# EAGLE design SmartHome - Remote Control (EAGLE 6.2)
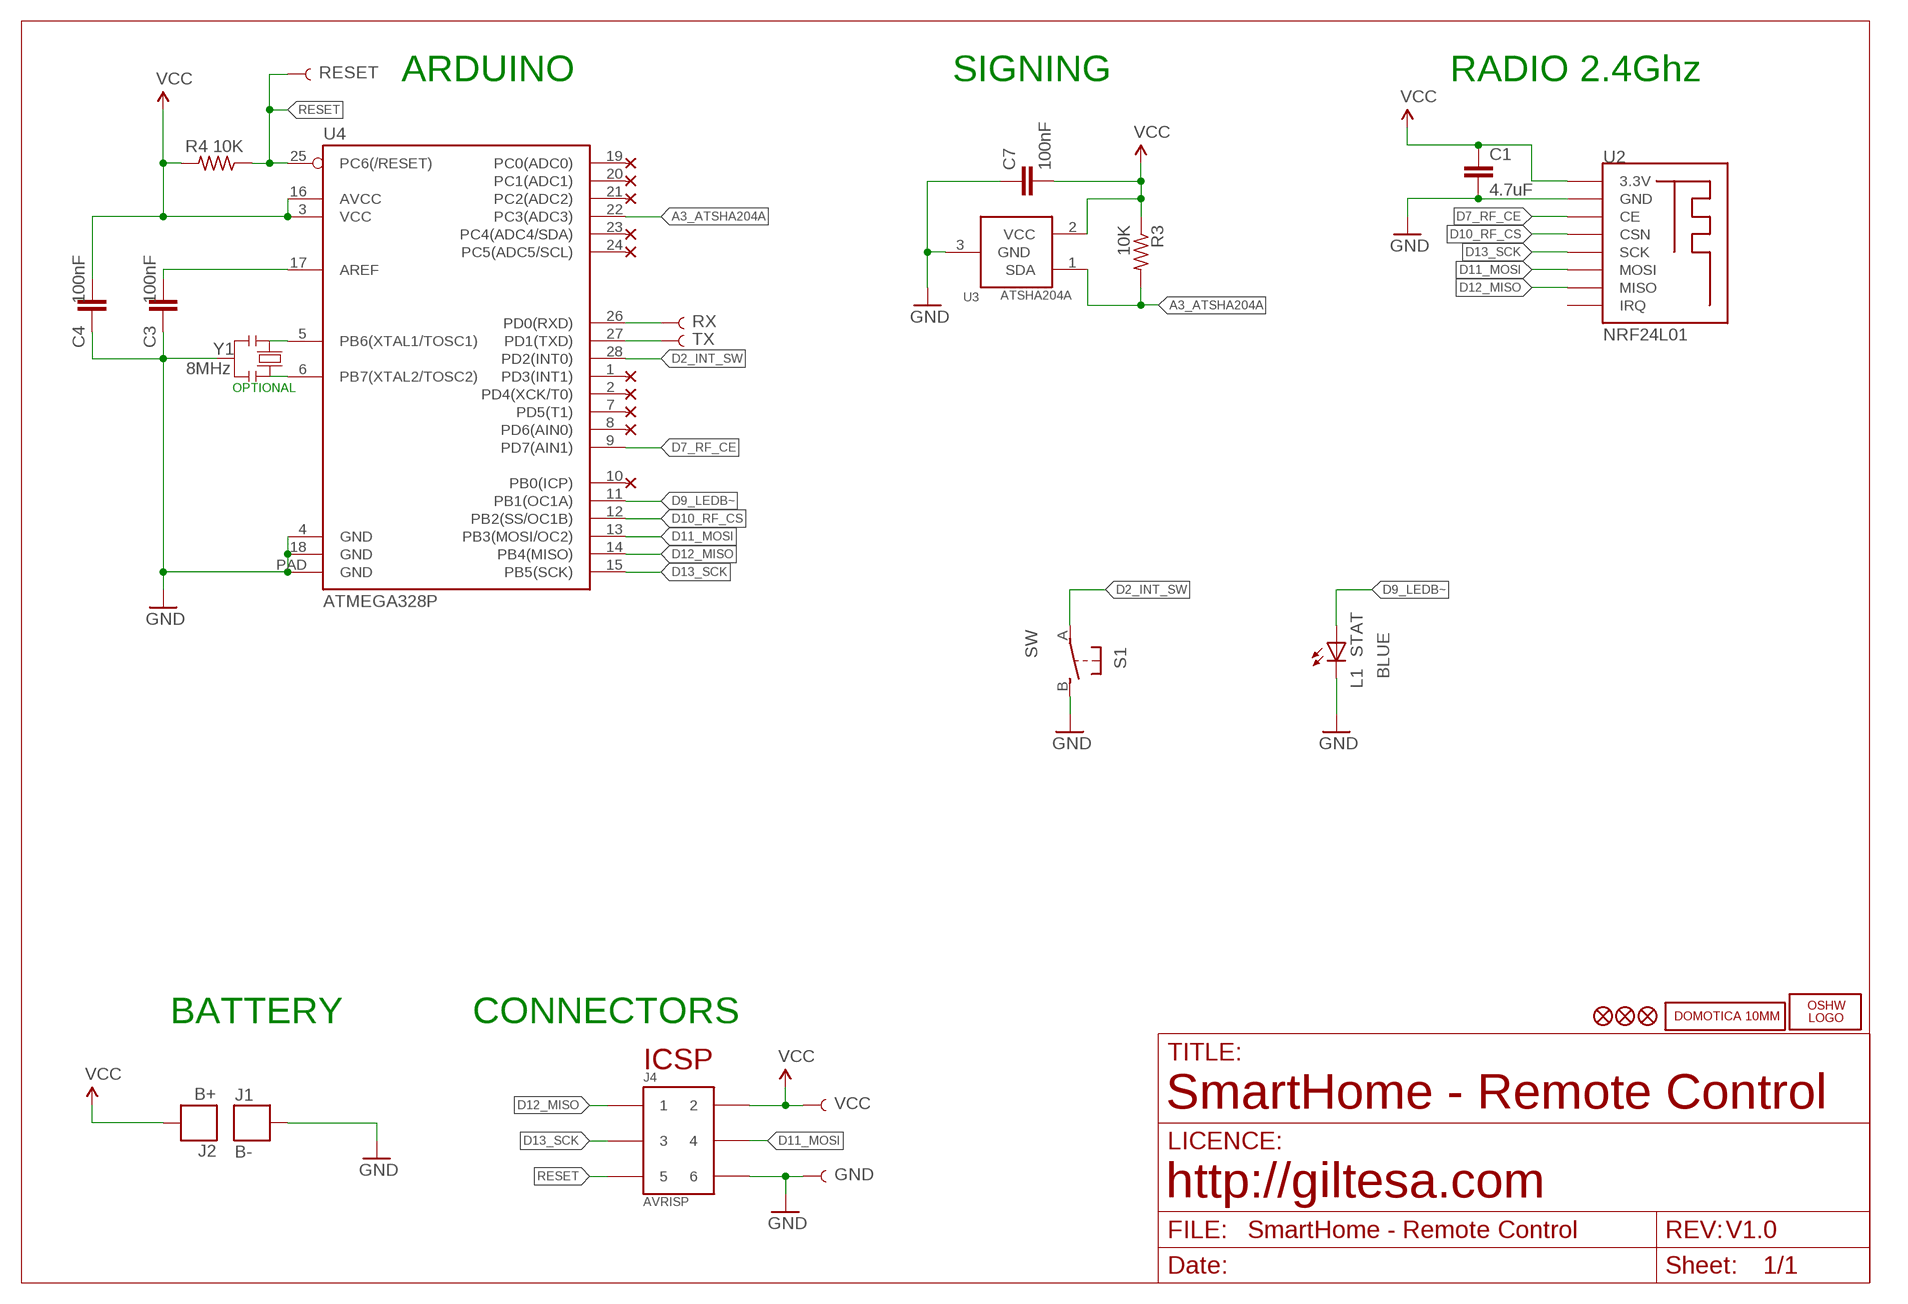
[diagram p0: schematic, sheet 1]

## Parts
C1  4.7uF  C1206  [C1206]
C3  100nF  C0603  [C0603]
C4  100nF  C0603  [C0603]
C7  100nF  C0603  [C0603]
J1  B-  PAD_KEYFINDER  [PAD_KEYFINDER]
J2  B+  PAD_KEYFINDER  [PAD_KEYFINDER]
J4  AVRISP  HEAD3X2  [HEAD3X2]
L1  STAT  LEDCHIP-LED0805  [CHIP-LED0805]
LOGO1  OSHW_LOGO_FILLX0150-NT  [OSHW_FILLX150_NOTEXT]
R3  10K  R0603  [R0603]
R4  10K  R0603  [R0603]
S1  SW  SWITCH-6X6MM-SMD  [SWITCH-6X6MM-SMD]
TP1  RX  TEST-POINT3  [PAD.03X.03]
TP2  TX  TEST-POINT3  [PAD.03X.03]
TP3  RESET  TEST-POINT3  [PAD.03X.03]
TP4  VCC  TEST-POINT3  [PAD.03X.03]
TP5  GND  TEST-POINT3  [PAD.03X.03]
U2  NRF24L01  NRF24L01_SMD  [NRF24L01_SMD]
U3  ATSHA204A  IC_ATSHA204A_CRYPT  [SOT23-3]
U4  ATMEGA328P  ATMEGA328P_VQFNVQFN  [VQFN-28]
U$5  DOMOTICA-10MM  [DOMOTICA-10MM]
U$6  FIDUCIAL1X2  [FIDUCIAL-1X2]
U$7  FIDUCIAL1X2  [FIDUCIAL-1X2]
U$14  FIDUCIAL1X2  [FIDUCIAL-1X2]
Y1  8MHz  RESONATORMU  [RESONATOR]

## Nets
A3_ATSHA204A: R3.2 U3.1(SDA) U4.22(PC3(ADC3))
D2_INT_SW: S1.A U4.28(PD2(INT0))
D7_RF_CE: U2.CE U4.9(PD7(AIN1))
D9_LEDB~: L1.A U4.11(PB1(OC1A))
D10_RF_CS: U2.CSN U4.12(PB2(SS/OC1B))
D11_MOSI: J4.4 U2.MOSI U4.13(PB3(MOSI/OC2))
D12_MISO: J4.1 U2.MISO U4.14(PB4(MISO))
D13_SCK: J4.3 U2.SCK U4.15(PB5(SCK))
GND [gnd]: C1.2 C3.1 C4.1 C7.1 J1.P$2 J4.6 L1.C S1.B TP5.P$1 U2.GND U3.3(GND) U4.4(GND) U4.18(GND) U4.PAD(GND) Y1.2
N$1: TP1.P$1 U4.26(PD0(RXD))
N$2: TP2.P$1 U4.27(PD1(TXD))
N$29: U4.5(PB6(XTAL1/TOSC1)) Y1.1
N$30: U4.6(PB7(XTAL2/TOSC2)) Y1.3
N$33: C3.2 U4.17(AREF)
RESET: J4.5 R4.1 TP3.P$1 U4.25(PC6(/RESET))
VCC: C1.1 C4.2 C7.2 J2.P$2 J4.2 R3.1 R4.2 TP4.P$1 U2.3.3V U3.2(VCC) U4.3(VCC) U4.16(AVCC)
Unconnected: U2.IRQ U4.1(PD3(INT1)) U4.2(PD4(XCK/T0)) U4.7(PD5(T1)) U4.8(PD6(AIN0)) U4.10(PB0(ICP)) U4.19(PC0(ADC0)) U4.20(PC1(ADC1)) U4.21(PC2(ADC2)) U4.23(PC4(ADC4/SDA)) U4.24(PC5(ADC5/SCL))

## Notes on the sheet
- ARDUINO | SIGNING | RADIO 2.4Ghz
- OPTIONAL
- BLUE
- BATTERY | CONNECTORS
- ICSP
- SmartHome - Remote Control
- http://giltesa.com
- V1.0

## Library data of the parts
C1 = ,giltesa:C1206
C3 C4 C7 = ,giltesa:C0603
J1 J2 = ,giltesa:PAD_KEYFINDER
J4 = MyCON2:HEAD3X2
L1 = led:LED: LED
LOGO1 = ohw-logo:OSHW_LOGO_FILL
R3 R4 = ,giltesa:R0603
S1 = ,giltesa:SWITCH-6X6MM-SMD
TP1-TP5 = SparkFun-Connectors:TEST-POINT: SparkFun Test Points
U2 = ,giltesa:NRF24L01_SMD
U3 = TD-MySensors:IC_ATSHA204A_CRYPT
U4 = SparkFun-IC-Microcontroller:ATMEGA328P_VQFN: Atmel 328P QFN part not in catalog
U$5 = ,giltesa_logos:DOMOTICA-10MM
U$6 U$7 U$14 = SparkFun:FIDUCIAL: Fiducial Alignment Points
Y1 = MySMD2:RESONATOR

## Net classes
2 gnd: width 0.305 mm, drill 0.406 mm, clearance 0.203 mm
3 usbvcc: width 0.203 mm, drill 0.406 mm, clearance 0.203 mm
4 USBpair: width 0.254 mm, drill 0.406 mm, clearance 0.61 mm

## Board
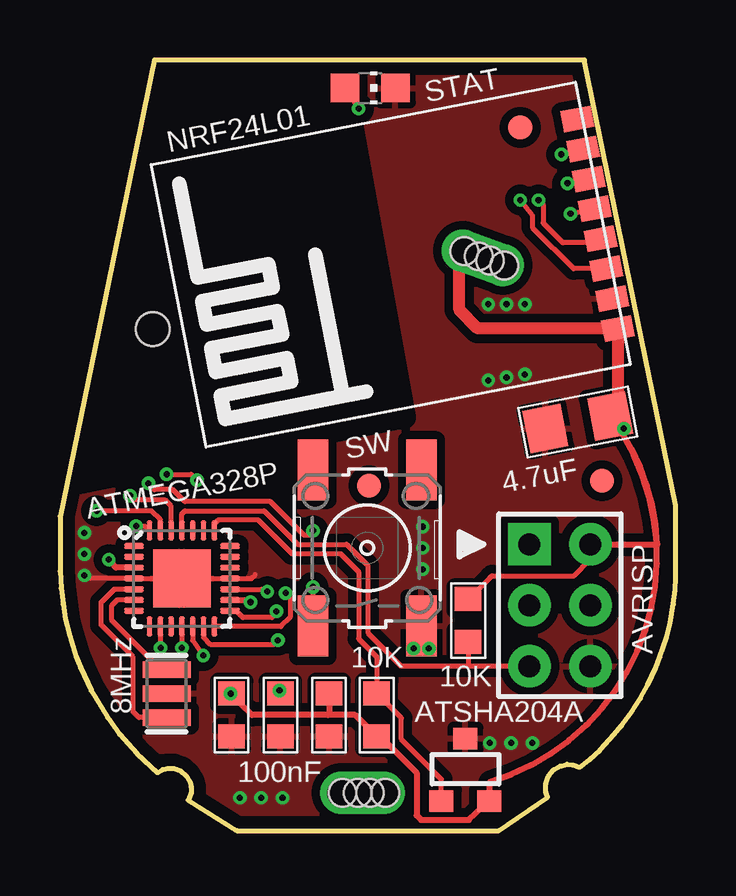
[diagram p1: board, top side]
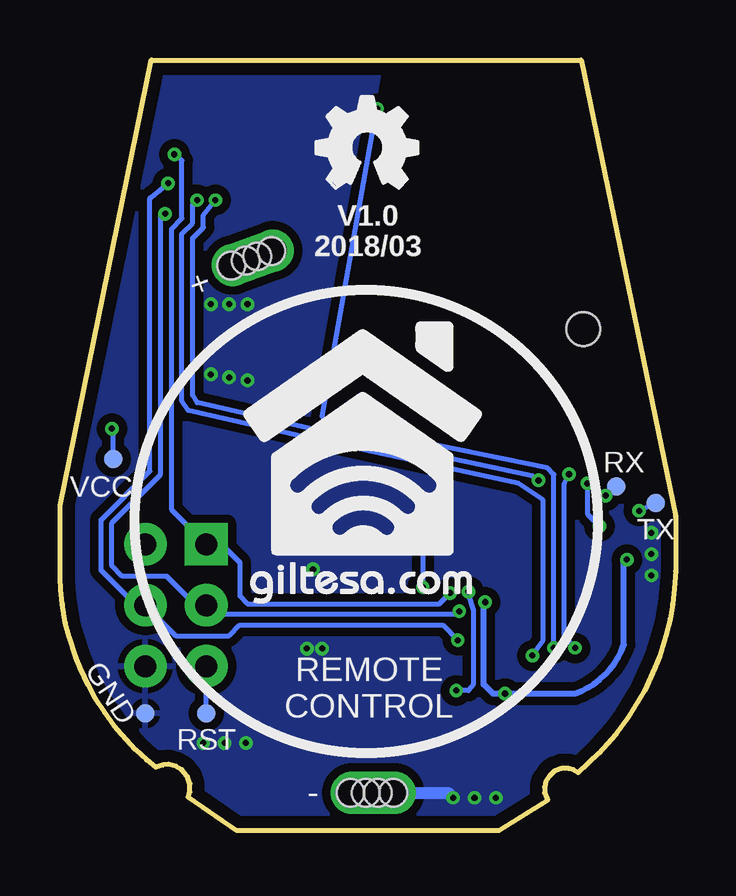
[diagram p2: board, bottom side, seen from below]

Size 25.65 x 32.13 mm. Coordinates in mm from the lower left corner, seen from the top.
Outline: 7.37,0 18.29,0 20.32,1.4 20.24,1.6 20.24,1.96 20.34,2.26 20.57,2.54 20.83,2.69 21.13,2.77 21.36,2.74 21.67,2.64 22.05,2.95 22.5,3.38 23.09,4.01 23.39,4.37 23.8,4.93 24.18,5.51 24.49,6.07 24.82,6.78 24.99,7.24 25.27,8.08 25.43,8.66 25.55,9.45 25.63,10.03 25.65,10.57 25.65,13.56 21.84,32.13 3.94,32.13 0,13.11 0,10.82 0.05,10.11 0.13,9.45 0.23,8.84 0.41,8.13 0.66,7.29 0.86,6.78 1.29,5.84 1.98,4.72 2.49,4.01 3.2,3.23 4.06,2.41 4.27,2.54 4.47,2.59 4.75,2.59 5.03,2.49 5.26,2.29 5.41,2.06 5.46,1.83 5.46,1.57 5.33,1.27 7.37,0
Copper layers (1*16): Top 0.035mm / dielectric 1.6mm / Bottom 0.035mm
Design rules: minimum track width 6mil, minimum drill 12mil, track to track 6mil, track to pad 6mil, pad to pad 6mil, via to via 8mil, smd to smd 0mil, copper to edge 20mil, drill to drill 10mil, minimum pad ring 6mil, minimum via ring 6mil, stop-mask expansion 0mil, vias tented up to drill 100mil, thermal gap 10mil
Holes 1.4 mm at 3.86,20.9
tRestrict: 4 lines
bRestrict: 4 lines

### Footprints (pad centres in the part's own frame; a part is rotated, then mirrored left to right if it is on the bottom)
C1206 = smd 1.6 x 1.8: 1 -1.362,-0.013; 2 1.387,-0.013
C0603 = smd 1 x 1.1: 1 -0.901,-0.038; 2 0.901,-0.038
PAD_KEYFINDER = drill 1.143 pad 1.778 offset: P$2 -0.889,0; P$3 0.889,0 | hole 1.143: -0.191,0; 0.318,0; -0.826,0; 0.953,0
HEAD3X2 = drill 0.914 pad 1.778 square: 1 0,0 | drill 0.914 pad 1.778: 2 0,2.54; 3 2.54,0; 4 2.54,2.54; 5 5.08,0; 6 5.08,2.54
CHIP-LED0805 = smd 1.2 x 1.2: A 0,-1.05; C 0,1.05
R0603 = smd 1 x 1.1: 1 -0.901,0.013; 2 0.901,0.013
SWITCH-6X6MM-SMD = smd 2.54 x 1.27: A -3.251,2.261; B -3.251,-2.261; NC@1 3.251,2.261; NC@2 3.251,-2.261
PAD.03X.03 = smd 0.762 x 0.762: P$1 0,0
NRF24L01_SMD = smd 0.9 x 1.27: 3.3V 1.575,0.203; CE 4.115,0.203; CSN 5.385,0.203; GND 2.845,0.203; IRQ 10.465,0.203; MISO 9.195,0.203; MOSI 7.925,0.203; SCK 6.655,0.203
SOT23-3 = smd 1 x 0.9: 1 -1,-1.3; 2 1,-1.3; 3 0,1.3
VQFN-28 = smd 0.82 x 0.24: 1 -2,1.35; 2 -2,0.9; 3 -2,0.45; 4 -2,0; 5 -2,-0.45; 6 -2,-0.9; 7 -2,-1.35; 15 2,-1.35; 16 2,-0.9; 17 2,-0.45; 18 2,0; 19 2,0.45; 20 2,0.9; 21 2,1.35 | smd 0.24 x 0.82: 8 -1.35,-2; 9 -0.9,-2; 10 -0.45,-2; 11 0,-2; 12 0.45,-2; 13 0.9,-2; 14 1.35,-2; 22 1.35,2; 23 0.9,2; 24 0.45,2; 25 0,2; 26 -0.45,2; 27 -0.9,2; 28 -1.35,2 | smd 2.4 x 2.4: PAD 0,0
FIDUCIAL-1X2 = smd 1 x 1: 1 0,0
RESONATOR = smd 0.7 x 2: 1 -1,0; 2 0,0; 3 1,0

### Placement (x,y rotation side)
C1  21.59,17.02 191 top
C3  9.14,4.83 90 top
C4  7.11,4.83 90 top
C7  11.18,4.83 90 top
J1  12.6,1.57 0 top
J2  17.62,23.88 340 top
J4  19.56,11.94 270 top
L1  12.93,30.96 270 top
LOGO1  14.99,26.8 0 bottom
R3  13.21,4.83 90 top
R4  17.02,8.76 90 top
S1  12.8,11.79 90 top
TP1  2.48,14.35 0 bottom
TP2  0.83,13.65 0 bottom
TP3  19.56,4.89 0 bottom
TP4  23.43,15.49 0 bottom
TP5  22.1,4.89 0 bottom
U2  23.75,19.43 101 top
U3  16.89,2.54 0 top
U4  5.08,10.52 0 top
U$5  18.03,9.4 0 bottom
U$6  12.88,14.38 0 top
U$7  19.18,29.31 0 top
U$14  22.58,14.58 0 top
Y1  4.45,5.71 90 top

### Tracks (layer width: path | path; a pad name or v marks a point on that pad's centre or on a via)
A3_ATSHA204A
  Top 0.203: U3.1 15.89,2.14 14.22,3.81 14.22,4.7 R3.2 13.21,7.24 12.45,8 12.45,10.79 11.68,11.56 9.65,11.56 8.26,12.95 6.6,12.95 6.43,12.78 U4.22
D2_INT_SW  (via drill 0.25)
  Top 0.203: v10.54,12.51 10.41,12.32 10.16,12.32 8.76,13.72 5.21,13.72 4.7,14.22 3.94,14.22 v3.68,14.48 | v10.54,10.16 S1.A | v3.17,12.7 3.55,12.7 U4.28
  Bottom 0.203: v10.54,12.51 v10.54,10.16 | v3.68,14.48 3.68,13.21 v3.17,12.7
D7_RF_CE  (via drill 0.25)
  Top 0.203: U4.9 v4.18,7.63 v4.19,7.62 | v4.45,14.86 5.46,14.86 v5.71,14.61 | 22.7,23.37 U2.CE 21.4,23.43 19.68,25.15 19.68,25.65 v19.18,26.29
  Bottom 0.203: v4.19,7.62 4.64,8.13 4.64,14.48 v4.45,14.86 | v5.71,14.61 5.97,14.8 14.99,16.7 19.94,17.84 20.13,18.16 20.13,24.7 19.68,25.15 19.68,25.65 v19.18,26.29
D9_LEDB~  (via drill 0.25)
  Top 0.203: U4.11 v5.08,7.62 | v12.45,30.1 L1.A
  Bottom 0.203: v5.08,7.62 5.08,14.86 5.33,15.11 14.61,17.02 14.73,17.27 v12.45,30.1
D10_RF_CS  (via drill 0.25)
  Top 0.203: U4.12 5.53,7.93 v5.97,7.3 | v19.94,26.29 20.13,26.1 20.13,25.34 20.95,24.51 22.1,24.51 22.31,24.72 22.31,24.89 U2.CSN
  Bottom 0.203: v5.97,7.3 5.52,7.94 5.52,13.78 6.54,14.48 15.37,16.38 20.32,17.53 20.57,17.91 20.57,24.89 20.13,25.34 20.13,26.1 v19.94,26.29
D11_MOSI  (via drill 0.25)
  Top 0.203: 22.1,27.18 22.1,27.11 U2.MOSI v21.14,26.99 | v9.08,7.94 8.89,7.75 6.29,7.75 5.98,8.05 U4.13
  Bottom 0.203: v21.14,26.99 21.84,26.42 21.91,26.35 21.91,14.99 23.94,12.95 23.94,10.86 22.48,9.4 J4.4 20.83,8.13 18.61,8.13 18.16,8.57 9.72,8.57 v9.08,7.94
D12_MISO  (via drill 0.25)
  Top 0.203: v20.89,28.19 U2.MISO | v9.4,9.91 9.59,9.72 9.59,8.89 9.21,8.51 U4.14
  Bottom 0.203: v20.89,28.19 20.57,27.94 20.57,25.53 21.02,25.08 21.02,13.4 J4.1 18.92,11.94 18.16,11.18 18.16,9.78 17.84,9.46 9.84,9.46 v9.4,9.91
D13_SCK  (via drill 0.25)
  Top 0.203: v21.27,25.72 U2.SCK | U4.15 7.34,9.17 7.62,8.89 8.83,8.89 v9.02,9.14
  Bottom 0.203: v21.27,25.72 21.46,25.59 21.46,14.86 23.5,12.83 23.5,11.05 23.05,10.6 21.21,10.6 20,9.4 J4.3 19.18,9.02 9.21,9.02 v9.02,9.14
GND  (via drill 0.25)
  Top 0.203: v1.02,10.64 1.14,10.52 U4.4 U4.PAD U4.18 7.98,10.52 8.13,10.67
  Bottom 0.406: 12.54,1.57 J1.P$2 11.65,1.57
  Bottom 0.508: 11.65,1.57 9.47,1.57 v9.27,1.37
  other vias: 17.91,3.66 18.8,3.66 19.68,3.66 7.49,1.37 8.38,1.37 1.02,12.42 1.02,11.53 15.11,10.9 15.11,11.79 15.11,12.67 19.37,19.02 18.61,18.9 17.84,18.77 17.84,21.95 18.61,21.95 19.37,21.95 14.73,7.59 15.37,7.59
  pour Bottom (isolate 0.356): 25.4,33.02 0,33.02 0,0 25.4,0
  pour Top (isolate 0.356): 0,33.02 25.4,33.02 25.4,0 0,0
N$1  (via drill 0.25)
  Top 0.203: U4.26 4.63,13.53 4.38,13.78 2.98,13.78 v2.92,13.97
  Bottom 0.203: v2.92,13.97 2.86,13.91 TP1.P$1
N$2  (via drill 0.25)
  Top 0.203: U4.27 4.18,12.96 3.81,13.34 v1.52,13.34
  Bottom 0.203: v1.52,13.34 TP2.P$1
N$29
  Top 0.203: U4.5 2.25,10.07 1.71,9.53 1.71,8.57 3.05,7.24 3.05,4.95 3.29,4.71 Y1.1
N$30
  Top 0.203: U4.6 2.38,9.62 2.16,9.4 2.16,8.76 4.21,6.71 Y1.3
N$33  (via drill 0.25)
  Top 0.203: U4.17 8.41,10.07 v8.64,9.97 | v9.14,5.84 9.17,5.84 C3.2
  Bottom 0.203: v8.64,9.97 8.64,9.84 8.45,9.21 8.45,6.1 8.64,5.84 v9.14,5.84
RESET
  Top 0.203: U4.25 5.08,13.21 5.21,13.34 8.51,13.34 9.91,11.94 11.94,11.94 12.83,11.05 12.83,8.26 14.22,6.86 17.02,6.86 | J4.5 17.02,6.86 | R4.1 17,6.87 17.02,6.86
  Bottom 0.203: TP3.P$1 J4.5
VCC  (via drill 0.25)
  Top 0.203: v7.11,5.71 7.16,5.84 C4.2 | R3.1 13.22,4.05 | 11.21,4.86 11.18,4.83 | R4.2 17.91,10.54 18,10.63 21.43,10.63 22.1,11.3 J4.2 | v23.5,16.76 23.45,16.76 C1.1
  Top 0.254: U4.16 7.91,9.62 v7.94,9.53 | C4.2 7.53,5.3 8,4.83 11.18,4.83 12.29,4.83 R3.1 | 13.22,4.05 14.86,2.41 14.86,0.64 15.05,0.45 17.03,0.45 U3.2 17.91,2.03 arc110 C1.1 arc-35 24.89,11.94 J4.2 | C7.2 11.21,4.86 | U4.3 2.33,10.97 v2.03,11.3 | 16.73,24.2 16.76,24.2 J2.P$2
  Top 0.406: 17.56,23.9 16.73,23.9 16.73,24.2
  Top 0.508: C1.1 arc90 23.25,17.61 U2.3.3V 17.42,20.94 16.64,21.72 16.64,24.12 16.73,24.2
  Bottom 0.203: TP4.P$1 23.43,16.7 v23.5,16.76
  Bottom 0.254: 7.94,9.59 v7.94,9.53 8,9.46 8,6.1 7.62,5.71 v7.11,5.71 4.19,5.71 arc-50 2.16,7.75 2.16,11.18 v2.03,11.3

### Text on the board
bPlace: V1.0 | 2018/03 | + | RX | VCC | TX | REMOTE | GND | CONTROL | RST | -

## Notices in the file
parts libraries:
SparkFun-IC-Microcontroller: Licensing: Creative Commons ShareAlike 4.0 International - https://creativecommons.org/licenses/by-sa/4.0
